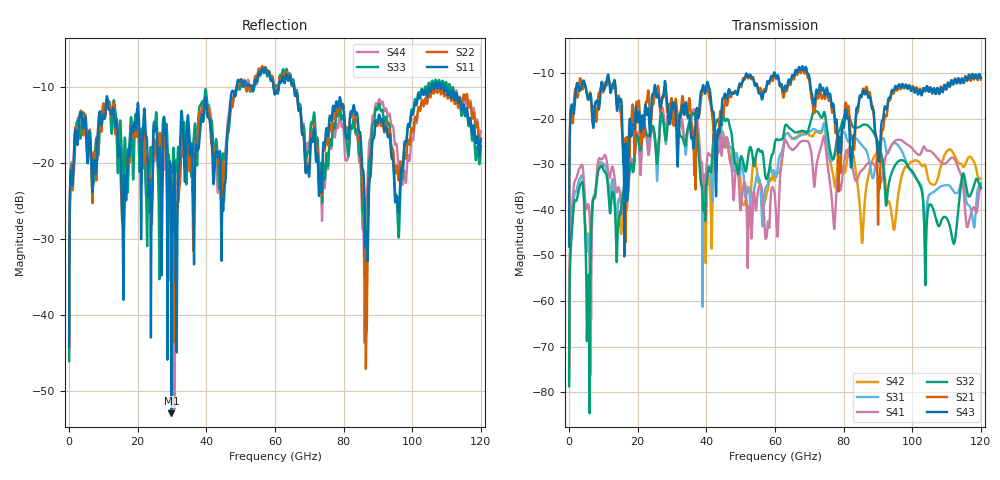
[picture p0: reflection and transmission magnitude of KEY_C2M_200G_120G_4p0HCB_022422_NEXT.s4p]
! Touchstone file
!  Generated:  6:09:51 AM  Oct 19, 2021
!  Setup:  LinearFrequency
!  Solution:  LinearFrequency
# GHz S MA R 50.000000
! Terminal data exported
! Port[1] = P2
! Port[2] = P4
! Port[3] = P6
! Port[4] = P8
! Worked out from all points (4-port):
!   12000 points, 10 MHz to 120 GHz, reference 50 ohm
!   strongest paths, dB at 10 MHz, 30.01 GHz, 60.01 GHz, 90.01 GHz, 120 GHz:
!     S43: -48.1, -16.5, -10.2, -27.7, -11.1
!     S21: -46.9, -16.1, -10.4, -42.2, -11.5
!     S32: -78.7, -17.8, -25.2, -25.3, -35.2
!     S41: -74.5, -16.7, -37.3, -32.7, -34.4
!     S31: -77.0, -16.8, -32.3, -27.2, -34.1
!     S42: -76.9, -17.4, -33.4, -27.7, -33.2
!   lowest |S11| = -53.0 dB at 29.8 GHz (marker M1), VSWR 1.00, Z = 50.1 - j0.185 ohm
!   |S11| at or under -10 dB: start of sweep to 48.84 GHz; 65.51 GHz to 105.6 GHz (40.1 GHz wide, 46.9 % of centre); 109.9 GHz to end of sweep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
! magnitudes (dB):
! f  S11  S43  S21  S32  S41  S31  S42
! 10 MHz  -44.2  -48.1  -46.9  -78.7  -74.5  -77.0  -76.9
! 3.12 GHz  -13.6  -13.9  -11.4  -34.8  -30.8  -33.3  -33.3
! 5.59 GHz  -18.7  -15.8  -15.7  -54.2  -38.8  -45.6  -45.2
! 8.91 GHz  -13.2  -16.7  -14.2  -30.8  -28.7  -29.6  -30.0
! 29.8 GHz  -53.0  -18.0  -15.6  -17.8  -17.0  -16.7  -17.6
! 57.5 GHz  -7.9  -13.2  -13.2  -33.3  -46.1  -34.9  -36.6
! 120 GHz  -16.9  -11.1  -11.5  -35.2  -34.4  -34.1  -33.2
